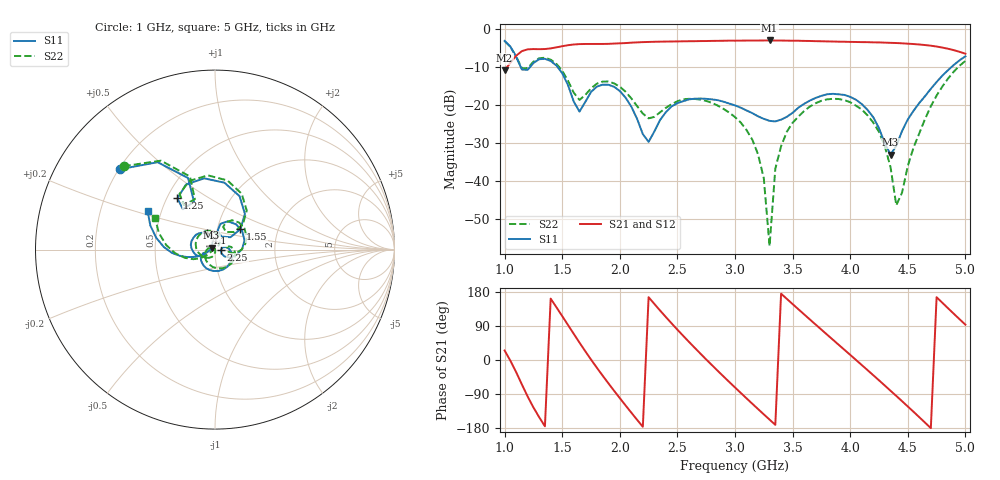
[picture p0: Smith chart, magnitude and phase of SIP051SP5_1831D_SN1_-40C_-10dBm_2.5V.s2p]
# GHz  S  dB  R  50
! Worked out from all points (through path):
!   81 points, 1 GHz to 5 GHz, reference 50 ohm
!   highest |S21| = -3.09 dB at 3.3 GHz (marker M1); lowest = -11.0 dB at 1 GHz (marker M2)
!   lowest |S11| = -33.1 dB at 4.35 GHz (marker M3), VSWR 1.05, Z = 48.1 + j1.06 ohm
!   |S11| at or under -10 dB: 1.139 GHz to 1.223 GHz (83.99 MHz wide, 7.11 % of centre); 1.458 GHz to 4.882 GHz (3.425 GHz wide, 108 % of centre)
!   |S22| runs from -57.2 to -3.2 dB; largest |S21 - S12| = 0.0023
!   S11 on the Smith chart (normalised r, x): 1 GHz: 0.21, +0.35; 1.25 GHz: 0.57, +0.37; 1.55 GHz: 1.29, +0.30; 2.25 GHz: 1.07, -0.00; 4.1 GHz: 0.90, +0.16; 5 GHz: 0.42, +0.22
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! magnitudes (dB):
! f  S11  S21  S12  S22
! 1 GHz  -3.2  -11.0  -11.0  -3.2
! 1.15 GHz  -10.7  -5.9  -5.9  -10.4
! 1.25 GHz  -9.0  -5.4  -5.4  -8.7
! 1.55 GHz  -14.8  -4.3  -4.3  -13.7
! 1.65 GHz  -21.8  -4.0  -4.0  -18.7
! 1.7 GHz  -19.3  -4.0  -4.0  -17.4
! 1.95 GHz  -15.3  -3.9  -3.9  -14.4
! 2.25 GHz  -29.8  -3.5  -3.5  -23.6
! 2.35 GHz  -24.0  -3.4  -3.4  -22.0
! 2.65 GHz  -18.4  -3.3  -3.3  -18.5
! 3 GHz  -20.2  -3.1  -3.1  -23.3
! 3.2 GHz  -23.1  -3.1  -3.1  -33.0
! 3.25 GHz  -23.7  -3.1  -3.1  -39.4
! 3.3 GHz  -24.2  -3.1  -3.1  -57.2
! 3.35 GHz  -24.4  -3.1  -3.1  -36.8
! 3.4 GHz  -23.9  -3.1  -3.1  -30.9
! 3.7 GHz  -18.2  -3.3  -3.3  -19.6
! 4.1 GHz  -19.8  -3.5  -3.5  -21.2
! 4.35 GHz  -33.1  -3.7  -3.7  -36.4
! 4.4 GHz  -30.8  -3.8  -3.8  -46.5
! 4.7 GHz  -15.8  -4.5  -4.5  -20.4
! 5 GHz  -7.3  -6.6  -6.6  -8.5
